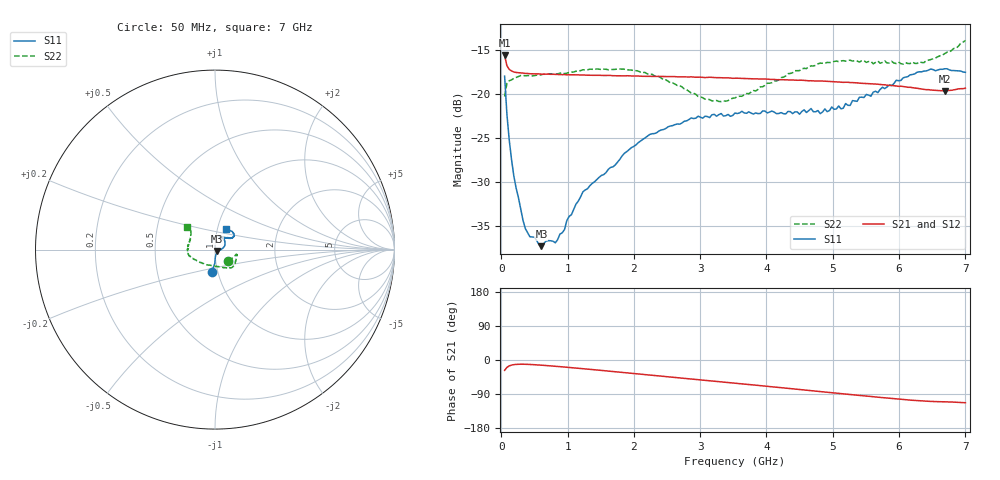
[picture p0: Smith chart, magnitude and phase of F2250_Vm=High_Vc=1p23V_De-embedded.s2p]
! Integrated Device Technology
! Corporate Headquarters
! 6024 Silver Creek Valley Road
! San Jose, CA 95138  USA
! Phone:  1-408-284-8200
! Toll Free:  1-800-223-1366
! Webpage:  http://www.idt.com/
! Timing and RF Division
! 515 Groton Road, Suite 102
! Westford, MA 01886-6024
! Device:  F2250
! Description: Voltage Variable RF Attenuator
! Frequency:  50.0 -  6000.00 MHz
! Package:  3x3 mm Thin QFN Plastic Package: 16 pin
! Ports:  2 RF, 3 DC
!  Pin  1  = GND
!  Pin  2  = NC
!  Pin  3  = RF1  = Port 1
!  Pin  4  = NC
!  Pin  5  = GND
!  Pin  6  = GND
!  Pin  7  = GND
!  Pin  8  = GND
!  Pin  9  = NC
!  Pin 10  = RF2  = Port 2
!  Pin 11  = NC
!  Pin 12  = GND
!  Pin 13  = GND
!  Pin 14  = VCNTRL
!  Pin 15  = VDD
!  Pin 16  = VMODE
! Vcntrl:  1.230 Volts
! Vmode:  +3.300 Volts
! Vdd:  +3.30  Volts
! Current:  1.332 mA
! Data:  The device was measured on a the F2250 evaluation board which has
!  individual transmission lines to the RF pins.  Data was collected
!  using a calibrated network analyzer.  The evaluation board was
!  de-embedded using a TRL calibration technique.
!  The reference plane is the edge of the package pin.
! Misc:  SN 10
!  Action Tracker AT0258
! Date Measured:  2014-11-26
! Date:  2015-10-15  MJV
! Note:
!  Integrated Device Technology supplies this data as a sample of measured
!  data at the package pin for this product.  Your particular data for this
!  product may vary.
!  Data was taken at 25 degrees C.
!  Integrated Device Technology reserves the right to change this data at anytime.
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# GHz S dB R 50
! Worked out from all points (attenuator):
!   201 points, 50 MHz to 7 GHz, reference 50 ohm
!   highest |S21| = -15.62 dB at 50 MHz (marker M1); lowest = -19.7 dB at 6.687 GHz (marker M2)
!   lowest |S11| = -37.3 dB at 606 MHz (marker M3), VSWR 1.03, Z = 51.1 - j0.81 ohm
!   |S11| at or under -10 dB: start of sweep to end of sweep
!   |S22| runs from -20.9 to -13.9 dB; largest |S21 - S12| = 0.00055
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0.05  -17.99 -98.2  -15.62 -27.2  -15.61 -27.2  -20.31 -40.8
0.08475  -22.32 -90.9  -16.80 -19.5  -16.81 -19.5  -18.81 -19.8
0.15425  -27.46 -87.6  -17.39 -13.5  -17.41 -13.5  -18.40 -12.6
0.189  -29.35 -84.1  -17.51 -12.3  -17.52 -12.3  -18.25 -12.2
0.328  -34.41 -64.8  -17.64 -11.1  -17.65 -11.1  -17.90 -12.9
0.43225  -36.27 -60.6  -17.71 -11.7  -17.70 -11.7  -17.93 -14.3
0.606  -37.33 -35.6  -17.77 -13.7  -17.75 -13.7  -17.81 -19.5
0.84925  -36.60 -19.8  -17.80 -17.0  -17.80 -17.0  -17.72 -26.3
1.2315  -31.14 -7.0  -17.85 -22.9  -17.85 -22.9  -17.26 -35.0
1.96125  -26.13 14.8  -17.96 -34.7  -17.95 -34.8  -17.29 -47.5
2.37825  -24.23 25.6  -18.01 -41.7  -18.01 -41.7  -18.02 -55.7
3.07325  -22.54 47.1  -18.15 -53.4  -18.12 -53.5  -20.60 -84.6
3.525  -22.18 60.7  -18.22 -61.2  -18.21 -61.2  -20.46 -116.2
4.7065  -22.03 66.9  -18.53 -81.4  -18.53 -81.4  -16.84 -164.7
5.15825  -21.63 50.0  -18.69 -89.2  -18.68 -89.3  -16.22 -173.9
5.193  -21.10 50.1  -18.68 -89.9  -18.68 -89.9  -16.27 -174.7
5.2625  -21.31 46.8  -18.72 -91.0  -18.71 -91.1  -16.17 -175.6
5.29725  -20.77 46.0  -18.72 -91.7  -18.72 -91.7  -16.27 -176.6
5.85325  -18.98 35.4  -19.04 -100.9  -19.03 -101.1  -16.48 169.9
6.3745  -17.41 37.6  -19.49 -108.3  -19.48 -108.4  -16.45 152.4
6.68725  -17.15 45.5  -19.67 -110.3  -19.66 -110.5  -15.42 142.3
7  -17.55 62.3  -19.35 -112.7  -19.35 -112.9  -13.92 140.3
